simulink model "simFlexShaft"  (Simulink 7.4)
settings: Solver=ode45  StartTime=0.0  StopTime=inf  RelTol=1e-3
InitFcn:
  | updateVarParamFlexShaft
StopFcn:
  | stopFcnFlexShaft
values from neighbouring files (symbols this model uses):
  cmd = 0    [initFcnFlexShaft.m]    (also in updateVarParamFlexShaft.m = 1)
  controllerSel = 0    [initFcnFlexShaft.m]    (also in updateVarParamFlexShaft.m)
  denzTfLoopShapingController = [1 1e-3*ones(1,3)]    [initFcnFlexShaft.m]    (also in updateVarParamFlexShaft.m = Grd.den{1,1})
  fcnSel = 0    [initFcnFlexShaft.m]    (also in updateVarParamFlexShaft.m = 2)
  feedbackGainObserver = 1e-3*ones(N,1)    [initFcnFlexShaft.m]    (also in updateVarParamFlexShaft.m = L)
  feedbackGainStateController = 1e-3*ones(1,N)    [initFcnFlexShaft.m]    (also in updateVarParamFlexShaft.m = K_bar(1,2:end))
  integralGainPidController = 0.0    (= 0)    [initFcnFlexShaft.m]    (also in updateVarParamFlexShaft.m)
  integralGainStateController = 0.0    (= 0)    [initFcnFlexShaft.m]    (also in updateVarParamFlexShaft.m = K_bar(1,1))
  numzTfLoopShapingController = 1e-3*ones(1,4)    [initFcnFlexShaft.m]    (also in updateVarParamFlexShaft.m = Grd.num{1,1})
  proportionalGainPidController = 0.0    (= 0)    [initFcnFlexShaft.m]    (also in updateVarParamFlexShaft.m)
  sysMatrixAcPlant = sysc.Ac    [initFcnFlexShaft.m]    (also in updateVarParamFlexShaft.m)
  sysMatrixAdObserver = sysd.a    [initFcnFlexShaft.m]    (also in updateVarParamFlexShaft.m = Ad)
  sysMatrixBcPlant = sysc.Bc    [initFcnFlexShaft.m]    (also in updateVarParamFlexShaft.m)
  sysMatrixBduObserver = sysd.b(:,1)    [initFcnFlexShaft.m]    (also in updateVarParamFlexShaft.m = Bd(:,1))
  sysMatrixCcPlant = sysc.Cc    [initFcnFlexShaft.m]    (also in updateVarParamFlexShaft.m)
  sysMatrixCdObserver = sysd.c    [initFcnFlexShaft.m]    (also in updateVarParamFlexShaft.m = Cd)
  sysMatrixDcPlant = sysc.Dc    [initFcnFlexShaft.m]    (also in updateVarParamFlexShaft.m)
undefined symbols (not defined in the file or in its folder): constParamFlexShaft
libraries: simulink x14, dspsnks4 x2, simulink_extras x1
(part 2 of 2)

== stateflow chart control/If Action
Subsystem1/refStepResp/controlStepSequenze ==
  state wait
    entry: stepVal=...
    stepSeq[idx][2];
  state terminated
    entry: fcnState=1;
  (default) -> wait : {idx=1; fcnState=0;}
  wait -> (junction 5) : [time>=... stepSeq[idx][1]]
  (junction 5) -> terminated : [idx>=nrOfSteps]
  (junction 5) -> wait : [idx<nrOfSteps]... {idx=idx+1;}

== stateflow chart control/If Action
Subsystem1/manipulatingFreqResp/controlSignalGenerator ==
  state delay
    entry: enFilter=0;
    during: krel=krel+1;
  state measure
    entry: enFilter=1;
    krel=nrOfSamplesDelay[idx]+1;
    during: krel=krel+1;
  state terminated
    entry: krel=0; enFilter=0;
    fcnState=1;
  delay -> measure : [krel==nrOfSamplesDelay[idx]]
  (default) -> delay : {idx=1; krel=0;... fcnState=0;}
  measure -> (junction 21) : [krel==nrOfSamplesFreq[idx]]
  (junction 21) -> terminated : [idx>=nrOfFreqs]
  (junction 21) -> delay : [idx<nrOfFreqs]... {idx=idx+1; krel=1;}

== stateflow chart control/If Action
Subsystem1/openLoopDistStepResp/controlStepSequenze ==
  state wait
    entry: stepVal=...
    stepSeq[idx][2];
  state terminated
    entry: fcnState=1;
  (default) -> wait : {idx=1; fcnState=0;}
  wait -> (junction 38) : [time>=... stepSeq[idx][1]]
  (junction 38) -> terminated : [idx>=nrOfSteps]
  (junction 38) -> wait : [idx<nrOfSteps]... {idx=idx+1;}

== stateflow chart control/If Action
Subsystem1/distFreqResp/controlSignalGenerator ==
  state delay
    entry: enFilter=0;
    during: krel=krel+1;
  state measure
    entry: enFilter=1;
    krel=nrOfSamplesDelay[idx]+1;
    during: krel=krel+1;
  state terminated
    entry: krel=0; enFilter=0;
    fcnState=1;
  delay -> measure : [krel==nrOfSamplesDelay[idx]]
  (default) -> delay : {idx=1; krel=0;... fcnState=0;}
  measure -> (junction 54) : [krel==nrOfSamplesFreq[idx]]
  (junction 54) -> terminated : [idx>=nrOfFreqs]
  (junction 54) -> delay : [idx<nrOfFreqs]... {idx=idx+1; krel=1;}

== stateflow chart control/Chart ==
  state idle
    entry: state=0; enable=0;
    reset=1;
    exit: reset=0;
  state running
    entry: state=1; enable=1;
    exit: enable=0;
  state failure
    entry: state=255;
  state terminated
    entry: state=2;
  (default) -> idle
  idle -> running : [cmd==1]
  running -> failure : [errorID>0]
  running -> idle : [cmd==0]
  failure -> idle : [cmd==0]
  running -> terminated : [fcnState==1]
  terminated -> idle : [cmd==0]
  terminated -> failure : [errorID>0]

== stateflow chart control/If Action
Subsystem1/closedLoopDistStepResp/controlStepSequenze ==
  state wait
    entry: stepVal1=stepSeq[idx][2];
    stepVal2=stepSeq[idx][3];
  state terminated
    entry: fcnState=1;
  (default) -> wait : {idx=1; fcnState=0;}
  wait -> (junction 91) : [time>=... stepSeq[idx][1]]
  (junction 91) -> terminated : [idx>=nrOfSteps]
  (junction 91) -> wait : [idx<nrOfSteps]... {idx=idx+1;}

== stateflow chart control/If Action
Subsystem1/manipulatingStepResp/controlStepSequenze ==
  state wait
    entry: stepVal=...
    stepSeq[idx][2];
  state terminated
    entry: fcnState=1;
  (default) -> wait : {idx=1; fcnState=0;}
  wait -> (junction 107) : [time>=... stepSeq[idx][1]]
  (junction 107) -> terminated : [idx>=nrOfSteps]
  (junction 107) -> wait : [idx<nrOfSteps]... {idx=idx+1;}

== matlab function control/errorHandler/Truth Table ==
function errorID = fcn(errorVector)

aVarTruthTableCondition_1 = false;
aVarTruthTableCondition_2 = false;
aVarTruthTableCondition_3 = false;
aVarTruthTableCondition_4 = false;
aVarTruthTableCondition_5 = false;
aVarTruthTableCondition_6 = false;
aVarTruthTableCondition_7 = false;
aVarTruthTableCondition_8 = false;
aVarTruthTableCondition_9 = false;
aVarTruthTableCondition_10 = false;


% modul not ok coder 1

aVarTruthTableCondition_1 = logical(errorVector(1) > 0);

% error 5VDC supply coder 1

aVarTruthTableCondition_2 = logical(errorVector(2) > 0);

% modul not ok power amplifier motor 1&2

aVarTruthTableCondition_3 = logical(errorVector(5) > 0);

% under voltage power amplifier motor 1&2

aVarTruthTableCondition_4 = logical(errorVector(6) > 0);

% over voltage power amplifier motor 1&2

aVarTruthTableCondition_5 = logical(errorVector(7) > 0);

% over temperature power amplifier motor 1&2

aVarTruthTableCondition_6 = logical(errorVector(8) > 0);

% current error power amplifier motor 1

aVarTruthTableCondition_7 = logical(errorVector(9) > 0);

% over current power amplifier motor 1

aVarTruthTableCondition_8 = logical(errorVector(10) > 0);

% current error power amplifier motor 2

aVarTruthTableCondition_9 = logical(errorVector(11) > 0);

% over current power amplifier motor 2

aVarTruthTableCondition_10 = logical(errorVector(12) > 0);

if (~aVarTruthTableCondition_1)
    aFcnTruthTableAction_1();
elseif (aVarTruthTableCondition_1 && aVarTruthTableCondition_2)
    aFcnTruthTableAction_2();
elseif (aVarTruthTableCondition_1 && ~aVarTruthTableCondition_2 && ~aVarTruthTableCondition_3)
    aFcnTruthTableAction_3();
elseif (aVarTruthTableCondition_1 && ~aVarTruthTableCondition_2 && aVarTruthTableCondition_3 && aVarTruthTableCondition_4)
    aFcnTruthTableAction_4();
elseif (aVarTruthTableCondition_1 && ~aVarTruthTableCondition_2 && aVarTruthTableCondition_3 && ~aVarTruthTableCondition_4 && aVarTruthTableCondition_5)
    aFcnTruthTableAction_5();
elseif (aVarTruthTableCondition_1 && ~aVarTruthTableCondition_2 && aVarTruthTableCondition_3 && ~aVarTruthTableCondition_4 && ~aVarTruthTableCondition_5 && aVarTruthTableCondition_6 && ~aVarTruthTableCondition_7 && ~aVarTruthTableCondition_8 && ~aVarTruthTableCondition_9 && ~aVarTruthTableCondition_10)
    aFcnTruthTableAction_6();
elseif (aVarTruthTableCondition_1 && ~aVarTruthTableCondition_2 && aVarTruthTableCondition_3 && ~aVarTruthTableCondition_4 && ~aVarTruthTableCondition_5 && aVarTruthTableCondition_7)
    aFcnTruthTableAction_7();
elseif (aVarTruthTableCondition_1 && ~aVarTruthTableCondition_2 && aVarTruthTableCondition_3 && ~aVarTruthTableCondition_4 && ~aVarTruthTableCondition_5 && ~aVarTruthTableCondition_7 && aVarTruthTableCondition_8)
    aFcnTruthTableAction_8();
elseif (aVarTruthTableCondition_1 && ~aVarTruthTableCondition_2 && aVarTruthTableCondition_3 && ~aVarTruthTableCondition_4 && ~aVarTruthTableCondition_5 && ~aVarTruthTableCondition_7 && ~aVarTruthTableCondition_8 && aVarTruthTableCondition_9)
    aFcnTruthTableAction_9();
elseif (aVarTruthTableCondition_1 && ~aVarTruthTableCondition_2 && aVarTruthTableCondition_3 && ~aVarTruthTableCondition_4 && ~aVarTruthTableCondition_5 && ~aVarTruthTableCondition_7 && ~aVarTruthTableCondition_8 && ~aVarTruthTableCondition_9 && aVarTruthTableCondition_10)
    aFcnTruthTableAction_10();
else % Default
    aFcnTruthTableAction_11();
end

function aFcnTruthTableAction_1()

% modul not ok coder 1

errorID=hex2dec('11');

function aFcnTruthTableAction_2()

% error 5VDC supply
% coder 1

errorID=hex2dec('12');

function aFcnTruthTableAction_3()

% modul not ok power amplifier motor 1&2

errorID=hex2dec('31');

function aFcnTruthTableAction_4()

% under voltage power amplifier motor 1&2

errorID=hex2dec('32');

function aFcnTruthTableAction_5()

% over voltage power amplifier motor 1&2

errorID=hex2dec('33');

function aFcnTruthTableAction_6()

% over temperature power amplifier motor 1&2

errorID=hex2dec('34');

function aFcnTruthTableAction_7()

% current error power amplifier motor 1

errorID=hex2dec('35');

function aFcnTruthTableAction_8()

% over current power amplifier motor 1

errorID=hex2dec('36');

function aFcnTruthTableAction_9()

% current error power amplifier motor 2

errorID=hex2dec('37');

function aFcnTruthTableAction_10()

% over current power amplifier motor 2

errorID=hex2dec('38');

function aFcnTruthTableAction_11()

% no error

errorID=hex2dec('00');
